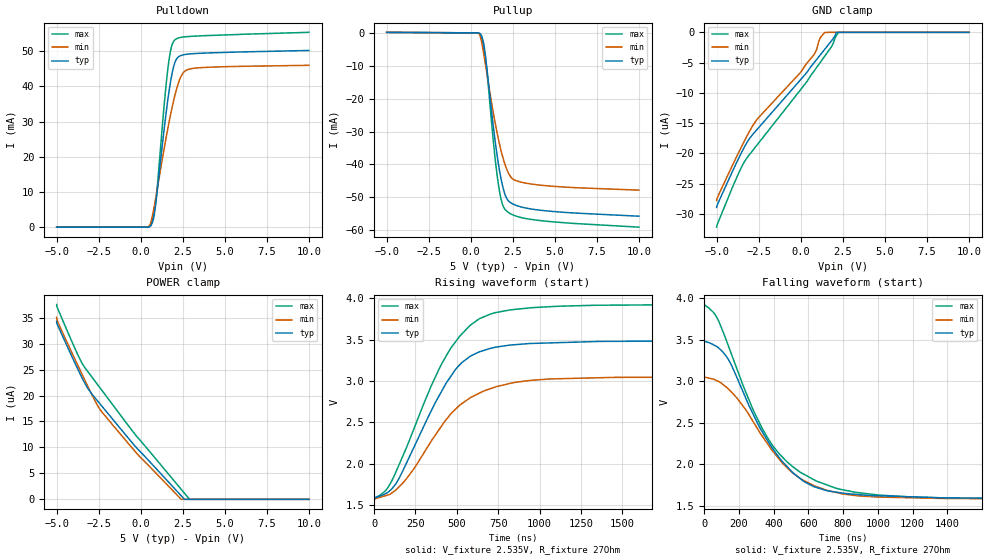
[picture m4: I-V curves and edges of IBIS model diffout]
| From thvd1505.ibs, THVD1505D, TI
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|   diffout Model
[Model]   diffout
Model_type   I/O
Polarity   Non-Inverting
Enable   Active-High
Vinl = 0.8
Vinh = 2
Vmeas = 2.5352
Vref = 2.5352
Cref = 50pF
Rref = 27
|   typ   min   max
C_comp   6.977pF   6.189pF   7.074pF
| Where Nom  PVT is Nominal Process, 5.0V, 25C
|   Fast PVT is Strong Process,  5.5V, -40C
|   Slow PVT is Weak Process,   4.5V, 150C
[Voltage Range]   5   4.5   5.5
|Junction Temperature
[Temperature Range]   25   150   -40
[Pullup Reference]   5   4.5   5.5
[Pulldown Reference]   0   0   -0
[Power Clamp Reference]   5   4.5   5.5
[GND Clamp Reference]   0   0   0
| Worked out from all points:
|   slope of the pulldown table from 0 to 0.75 V, typ, clamps not added: 336 ohm
|   slope of the pullup table from 0 to 0.75 V, typ, clamps not added: 274 ohm
|   falling waveform, V_fixture 2.535V, R_fixture 27Ohm: 20-80 % time 304ns typ, 319ns min, 334ns max; typ from 3.49 V to 1.58 V
|   rising waveform, V_fixture 2.535V, R_fixture 27Ohm: 20-80 % time 295ns typ, 336ns min, 321ns max; typ from 1.58 V to 3.49 V
[Pulldown]
|   Voltage   I(typ)   I(min)   I(max)
-5V       -16.79uA   -14.96uA   -18.63uA
295mV     -450.9nA   -235.1nA   8.726uA
580mV     300.3uA    1.014mA    453.7uA
745mV     2.115mA    4.385mA    3.115mA
910mV     7.308mA    8.762mA    7.985mA
1.405V    28.38mA    22.63mA    35.31mA
1.645V    37.34mA    28.88mA    46.2mA
1.855V    43.49mA    33.82mA    51.74mA
2.05V     47.05mA    37.82mA    53.35mA
2.515V    48.99mA    43.83mA    54.07mA
2.98V     49.29mA    45.04mA    54.25mA
10V       50.24mA    46.02mA    55.4mA
[GND Clamp]
|   Voltage   I(typ)   I(min)   I(max)
-5V       -28.92uA   -27.78uA   -32.19uA
-3.53V    -19.91uA   -18.95uA   -22.32uA
-3.095V   -17.76uA   -16.6uA    -20.37uA
-2.69V    -16.34uA   -14.73uA   -18.94uA
25mV      -7.717uA   -6.496uA   -9.356uA
820mV     -4.924uA   -3.559uA   -6.285uA
1.135V    -3.828uA   -1.062uA   -5.071uA
1.42V     -2.833uA   -29.56nA   -3.968uA
1.87V     -1.252uA   0A         -2.186uA
2.11V     -90.82nA   0A         -566.7nA
2.245V    0A         0A         -35.93nA
10V       0A         0A         0A
[Pullup]
|   Voltage   I(typ)   I(min)   I(max)
-5V       158.2uA    151.5uA    169uA
295mV     24.81uA    18.88uA    24.65uA
565mV     -274.7uA   -1.072mA   -407uA
760mV     -2.953mA   -5.95mA    -4.173mA
940mV     -9.88mA    -11.68mA   -10.47mA
1.36V     -29.15mA   -24.77mA   -33.72mA
1.645V    -39.79mA   -32.27mA   -46.03mA
1.9V      -46.64mA   -37.66mA   -52.3mA
2.185V    -50.74mA   -41.98mA   -54.39mA
2.53V     -52.08mA   -44.54mA   -55.4mA
3.655V    -53.6mA    -45.99mA   -56.76mA
10V       -55.74mA   -47.82mA   -59.07mA
[POWER Clamp]
|   Voltage   I(typ)   I(min)   I(max)
-5V       34.28uA    35.06uA    37.54uA
-4.955V   33.66uA    34.38uA    36.91uA
-4.595V   31.08uA    31.76uA    34.16uA
-3.545V   23.78uA    24.47uA    26.56uA
-3.17V    21.5uA     21.92uA    24.72uA
-2.63V    19.21uA    18.44uA    22.39uA
-2.315V   17.97uA    16.85uA    21.03uA
-140mV    9.55uA     8.512uA    11.77uA
2.395V    733.2nA    41.11nA    1.978uA
2.62V     0A         0A         1.105uA
2.89V     0A         0A         56.59nA
10V       0A         0A         0A
[Ramp]
R_load = 27
|   typ   min   max
dV/dt_r   1.14078/2.93774e-07   0.882388/3.32142e-07   1.40798/3.19711e-07
dV/dt_f   1.14078/3.02423e-07   0.882391/3.16279e-07   1.40799/3.33864e-07
[Falling Waveform]
V_fixture = 2.535V
V_fixture_min = 2.316V
V_fixture_max = 2.75V
R_fixture = 27Ohm
C_fixture = 0F
|   Time   V(typ)   V(min)   V(max)
0s        3.486V     3.051V     3.924V
66.57ns   3.427V     3.015V     3.795V
131.4ns   3.292V     2.925V     3.476V
275ns     2.636V     2.541V     2.692V
393.9ns   2.192V     2.162V     2.228V
569.3ns   1.8V       1.81V      1.885V
756.3ns   1.665V     1.662V     1.713V
1.002us   1.62V      1.604V     1.629V
1.422us   1.594V     1.587V     1.591V
4us       1.585V     1.58V      1.577V
[Rising Waveform]
V_fixture = 2.535V
V_fixture_min = 2.316V
V_fixture_max = 2.75V
R_fixture = 27Ohm
C_fixture = 0F
|   Time   V(typ)   V(min)   V(max)
0s        1.585V     1.58V      1.577V
72.1ns    1.642V     1.615V     1.681V
131.4ns   1.756V     1.681V     1.896V
346.6ns   2.642V     2.276V     2.945V
453.4ns   3.025V     2.575V     3.363V
579.2ns   3.295V     2.794V     3.668V
706.3ns   3.395V     2.909V     3.811V
948.2ns   3.453V     3.007V     3.885V
1.451us   3.479V     3.043V     3.916V
4us       3.486V     3.051V     3.924V
